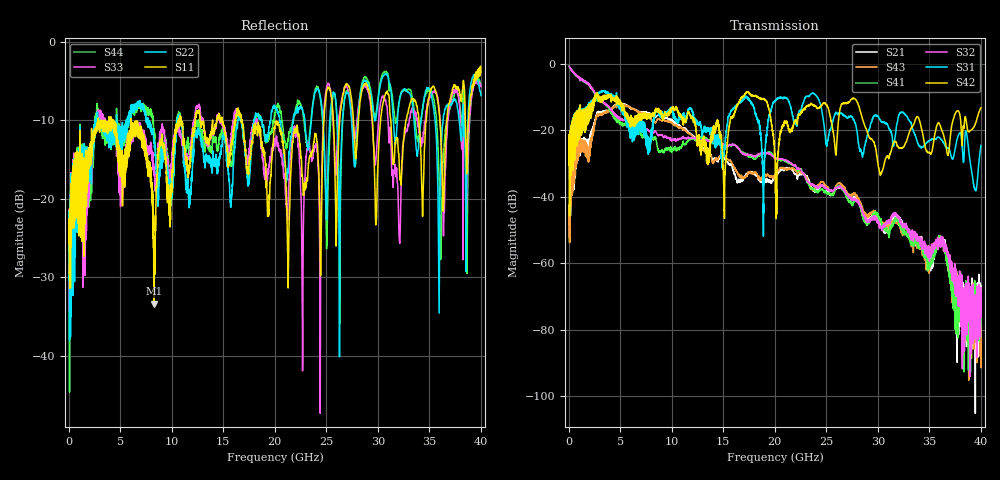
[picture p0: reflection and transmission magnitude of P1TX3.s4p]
!Agilent Technologies,N5245A,MY49151084,A.09.20.08
!Agilent N5245A: A.09.20.08
!Date: Thursday, March 01, 2012 10:49:01
!Correction: S11(Full 4 Port(1,2,3,4))
!S12(Full 4 Port(1,2,3,4))
!S13(Full 4 Port(1,2,3,4))
!S14(Full 4 Port(1,2,3,4))
!S21(Full 4 Port(1,2,3,4))
!S22(Full 4 Port(1,2,3,4))
!S23(Full 4 Port(1,2,3,4))
!S24(Full 4 Port(1,2,3,4))
!S31(Full 4 Port(1,2,3,4))
!S32(Full 4 Port(1,2,3,4))
!S33(Full 4 Port(1,2,3,4))
!S34(Full 4 Port(1,2,3,4))
!S41(Full 4 Port(1,2,3,4))
!S42(Full 4 Port(1,2,3,4))
!S43(Full 4 Port(1,2,3,4))
!S44(Full 4 Port(1,2,3,4))
!S4P File: Measurements: <S11,S12,S13,S14>,
!<S21,S22,S23,S24>,
!<S31,S32,S33,S34>,
!<S41,S42,S43,S44>:
# Hz S  dB  R 50
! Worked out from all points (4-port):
!   3996 points, 50 MHz to 40 GHz, reference 50 ohm
!   strongest paths, dB at 50 MHz, 10.04 GHz, 20.03 GHz, 30.02 GHz, 40 GHz:
!     S42: -25.4, -13.5, -27.7, -30.2, -13.2
!     S31: -25.3, -14.0, -11.2, -15.9, -24.6
!     S32: -0.7, -23.0, -28.3, -48.1, -67.5
!     S41: -0.8, -26.0, -28.1, -45.2, -78.7
!     S43: -44.8, -17.8, -33.2, -46.3, -71.8
!     S21: -44.0, -17.0, -33.7, -46.7, -66.7
!   lowest |S11| = -33.4 dB at 8.31 GHz (marker M1), VSWR 1.04, Z = 52.2 - j0.288 ohm
!   |S11| at or under -10 dB: start of sweep to 2.876 GHz; 6.042 GHz to 10.63 GHz (4.588 GHz wide, 55 % of centre); 16.83 GHz to 24.77 GHz (7.941 GHz wide, 38.2 % of centre)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
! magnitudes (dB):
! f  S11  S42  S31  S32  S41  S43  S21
! 50 MHz  -23.8  -25.4  -25.3  -0.7  -0.8  -44.8  -44.0
! 2.82 GHz  -10.8  -9.8  -9.2  -10.2  -10.7  -15.7  -14.9
! 8.31 GHz  -33.4  -15.1  -16.3  -20.5  -22.0  -17.5  -15.8
! 20.16 GHz  -10.2  -39.9  -10.8  -28.6  -28.5  -32.4  -33.6
! 27.7 GHz  -11.4  -10.4  -16.9  -40.7  -41.4  -39.1  -40.3
! 30.3 GHz  -9.6  -32.9  -17.3  -49.2  -47.4  -47.4  -47.8
! 40 GHz  -3.9  -13.2  -24.6  -67.5  -78.7  -71.8  -66.7
